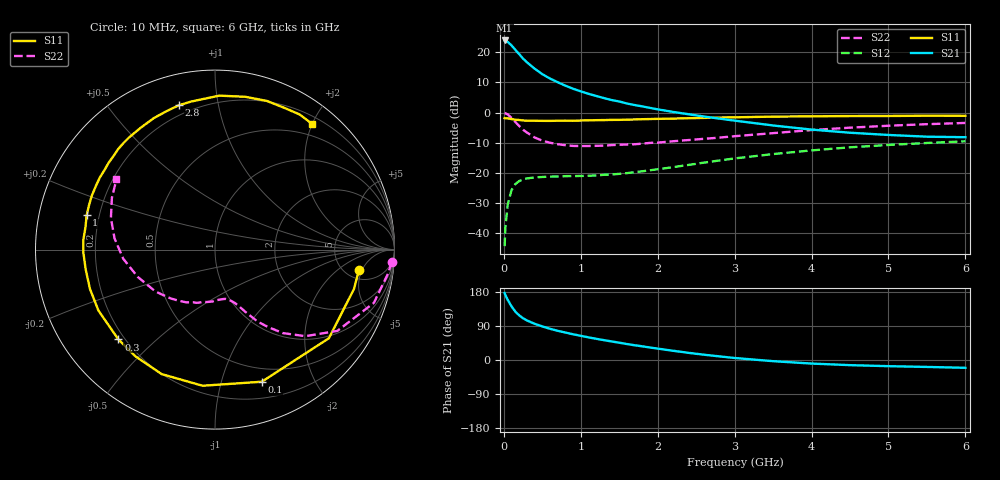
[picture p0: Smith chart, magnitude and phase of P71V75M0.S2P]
! SIEMENS Small Signal Semiconductors
! BFP196
! Si NPN RF Bipolar Junction Transistor in SOT143
! VCE = 1.75 V  IC = 5 mA
! Common Emitter S-Parameters:  May  1996
# GHz  S  MA  R  50
!  f  S11  S21  S12  S22
! GHz  MAG  ANG  MAG  ANG  MAG  ANG  MAG  ANG
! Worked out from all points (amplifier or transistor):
!   36 points, 10 MHz to 6 GHz, reference 50 ohm
!   highest |S21| = 23.9 dB at 10 MHz (marker M1)
!   |S21| within 3 dB of that: start of sweep to 145.8 MHz
!   unconditionally stable (mu >= 1): 1.096 GHz to 3.275 GHz; 5.783 GHz to end of sweep
!   at 250 MHz: K = 0.26, MSG = 20.0 dB, |S12| = -22.2 dB
!   at 1.4 GHz: K = 1.16, MAG = 10.0 dB, |S12| = -20.5 dB
!   at 6 GHz: K = 1.01, MAG = 0.2 dB, |S12| = -9.5 dB
!   S11 on the Smith chart (normalised r, x): 10 MHz: 6.63, -4.35; 100 MHz: 0.36, -1.35; 300 MHz: 0.18, -0.38; 1 GHz: 0.15, +0.13; 2.8 GHz: 0.15, +0.77; 6 GHz: 0.31, +2.00
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0.01  0.8101 -8.0  15.72 176.6  0.0061 86.0  0.9862 -4.0
0.02  0.8049 -15.8  15.52 171.2  0.0123 80.2  0.975 -7.6
0.05  0.8041 -37.9  14.89 159.0  0.0298 70.6  0.9338 -18.5
0.1  0.7809 -70.5  13.02 141.5  0.0519 55.8  0.8184 -33.6
0.15  0.7617 -95.2  10.97 127.5  0.0653 44.6  0.697 -43.8
0.2  0.7546 -113.2  9.311 117.8  0.0733 37.4  0.5992 -50.9
0.25  0.7417 -126.8  7.864 110.1  0.078 32.2  0.521 -55.7
0.3  0.7349 -137.1  6.834 104.4  0.081 28.9  0.4676 -59.3
0.4  0.7329 -152.4  5.362 95.6  0.0841 24.3  0.3875 -63.9
0.5  0.7303 -162.5  4.34 88.6  0.0857 21.8  0.3423 -67.1
0.6  0.7289 -171.3  3.674 82.4  0.0869 20.7  0.3167 -69.7
0.7  0.7338 -178.8  3.187 77.0  0.0871 20.4  0.2994 -72.6
0.9  0.7324 170.3  2.489 67.9  0.0887 21.4  0.2804 -78.2
1  0.7403 165.0  2.252 63.8  0.089 22.3  0.2792 -80.9
1.1  0.7443 160.5  2.051 59.8  0.0897 23.4  0.2796 -83.9
1.6  0.765 140.8  1.416 42.1  0.0993 31.1  0.2962 -99.6
2.2  0.7952 121.3  1.027 24.4  0.1247 37.8  0.3351 -118.8
2.8  0.8289 104.1  0.796 9.6  0.1607 38.1  0.3849 -138.9
3.5  0.8581 88.4  0.612 -3.1  0.2055 32.7  0.4569 -160.6
4.5  0.8773 70.8  0.464 -13.6  0.2658 21.5  0.563 173.7
5.5  0.8885 57.9  0.399 -18.3  0.3137 9.0  0.643 153.3
6  0.885 52.2  0.391 -20.6  0.3344 2.4  0.6746 144.5
